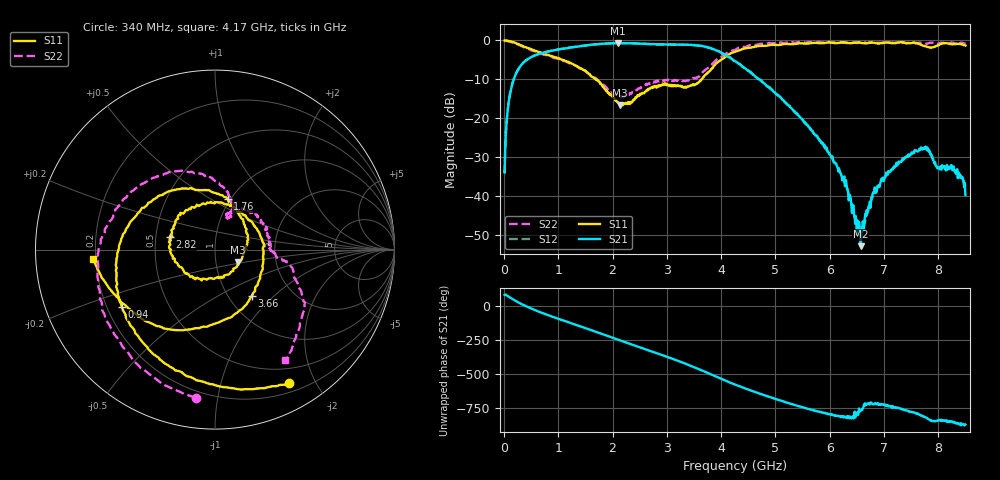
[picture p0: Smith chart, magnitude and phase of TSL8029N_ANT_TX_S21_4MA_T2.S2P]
!Agilent Technologies,E5071C,MY46523237,B.13.01
!Date: Tue Nov 14 09:47:55 2023
!Data & Calibration Information:
!Freq	S11:SOLT2(ON)	S21:SOLT2(ON)	S12:SOLT2(ON)	S22:SOLT2(ON)
!PortZ  Port1:50+j0  Port2:50+j0
!Above PortZ is port z conversion or system Z0 setting when saving the data.
!When reading, reference impedance value at option line is always used.
# Hz S dB R 50
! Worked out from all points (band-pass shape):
!   850 points, 10 MHz to 8.5 GHz, reference 50 ohm
!   highest |S21| = -0.64 dB at 2.1 GHz (marker M1); lowest = -52.8 dB at 6.57 GHz (marker M2)
!   |S21| within 3 dB of the highest: 602.4 MHz to 4.07 GHz (3.467 GHz wide, 148 % of centre)
!   lowest |S11| = -16.7 dB at 2.14 GHz (marker M3), VSWR 1.34, Z = 64.2 - j9.08 ohm
!   |S11| at or under -10 dB: 1.688 GHz to 3.637 GHz (1.948 GHz wide, 73.2 % of centre)
!   |S22| runs from -14.6 to 0.0 dB; largest |S21 - S12| = 0.021
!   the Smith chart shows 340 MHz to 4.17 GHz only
!   S11 on the Smith chart (normalised r, x): 340 MHz: 0.31, -1.65; 940 MHz: 0.26, -0.26; 1.76 GHz: 0.97, +0.60; 2.82 GHz: 0.59, +0.09; 3.66 GHz: 1.27, -0.74; 4.17 GHz: 0.19, -0.04
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1e7  0.00 -2.0  -33.73 80.3  -34.17 87.3  -0.03 -3.3
1.2e8  -0.25 -23.2  -13.03 59.3  -13.00 58.8  -0.37 -37.8
3.4e8  -1.40 -61.1  -5.95 10.1  -5.91 10.0  -1.59 -97.5
9.4e8  -4.30 -148.5  -2.48 -86.2  -2.49 -86.2  -4.45 158.2
1.43e9  -7.24 136.6  -1.43 -153.6  -1.39 -153.8  -7.34 100.6
1.76e9  -10.69 76.1  -0.89 160.5  -0.91 160.4  -10.66 71.8
2.1e9  -16.02 -10.6  -0.64 112.1  -0.69 112.2  -14.30 69.6
2.14e9  -16.66 -28.1  -0.67 106.7  -0.68 106.5  -14.30 69.1
2.82e9  -11.63 164.1  -1.00 11.4  -0.99 11.4  -10.48 39.5
2.84e9  -11.82 158.9  -0.97 8.5  -1.02 8.5  -10.34 38.6
3.33e9  -12.06 51.3  -1.11 -62.5  -1.10 -62.8  -10.41 3.4
3.66e9  -9.63 -52.0  -1.45 -116.4  -1.49 -116.5  -8.16 -9.0
4.17e9  -3.35 -175.7  -4.53 156.2  -4.41 157.5  -2.76 -57.6
4.26e9  -2.89 166.4  -5.34 141.3  -5.50 142.1  -2.41 -69.2
4.77e9  -1.41 73.5  -10.79 67.6  -10.83 69.7  -0.84 -123.7
5.19e9  -0.89 0.5  -15.98 12.3  -16.04 12.8  -0.60 -162.9
5.67e9  -0.68 -71.6  -23.11 -42.5  -23.10 -41.0  -0.44 157.1
6.57e9  -0.58 -170.2  -52.76 -48.1  -49.32 -44.9  -0.45 81.3
7.09e9  -0.55 135.6  -33.85 -13.5  -33.94 -15.3  -0.60 36.5
7.59e9  -0.61 75.8  -28.20 -70.6  -28.58 -69.8  -0.75 -8.1
8.13e9  -0.66 18.6  -32.52 -124.2  -32.34 -123.0  -0.78 -57.4
8.5e9  -1.30 -28.4  -39.65 -151.7  -37.40 -154.7  -0.86 -95.3
